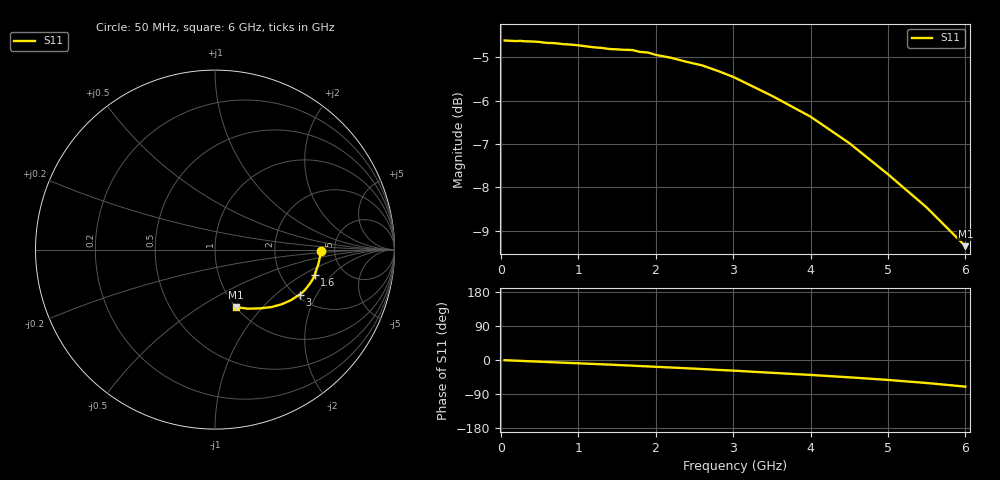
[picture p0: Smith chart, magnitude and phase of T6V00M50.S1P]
! SIEMENS Discrete & RF Semiconductors
! BAT62
! Si Schottky Diode in SOT143
! IF = 0.5 mA
! S-Parameters:  February  1997
# GHz  S  MA  R  50
!  f  S11
! GHz  MAG  ANG
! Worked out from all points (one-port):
!   34 points, 50 MHz to 6 GHz, reference 50 ohm
!   lowest |S11| = -9.4 dB at 6 GHz (marker M1), VSWR 2.03, Z = 49.9 - j36.2 ohm
!   |S11| at or under -10 dB: nowhere
!   S11 on the Smith chart (normalised r, x): 50 MHz: 3.85, -0.06; 1.6 GHz: 3.11, -1.28; 3 GHz: 2.09, -1.46; 6 GHz: 1.00, -0.72
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0.05  0.5879 -0.5
0.25  0.5873 -2.2
0.4  0.5864 -3.6
0.5  0.5856 -4.4
0.6  0.5841 -5.3
0.7  0.5838 -6.2
0.8  0.5823 -7.0
0.9  0.5815 -7.9
1  0.5804 -8.7
1.3  0.5765 -11.3
1.4  0.5748 -12.1
1.5  0.5742 -13.1
1.6  0.5735 -14.0
1.7  0.5732 -14.9
1.8  0.5703 -16.0
1.9  0.5695 -16.8
2  0.5659 -18.0
2.2  0.5615 -19.8
2.4  0.5555 -21.8
2.6  0.5503 -23.8
2.8  0.5423 -26.1
3  0.5338 -28.0
3.5  0.5077 -33.8
4  0.4803 -39.4
4.5  0.4477 -45.7
5  0.4122 -52.6
5.5  0.3774 -60.7
6  0.3405 -70.3
